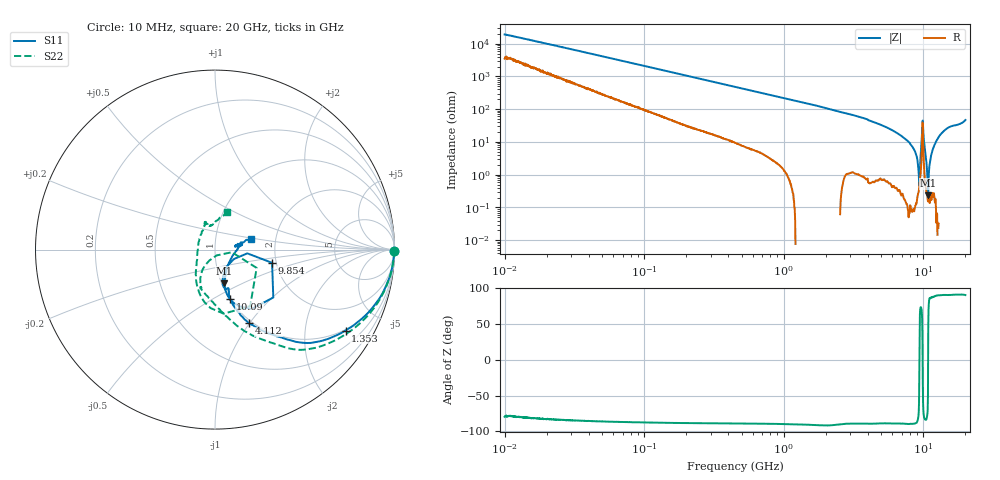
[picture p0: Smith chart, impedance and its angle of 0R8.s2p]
!Keysight Technologies,P5008B,MY61100088,A.16.20.02
!Date: Monday, October 30, 2023 15:59:24
!Correction: S11(C  2-Port  )
!S21(C  2-Port  )
!S12(C  2-Port  )
!S22(C  2-Port  )
!S2P File: Measurements: S11, S21, S12, S22:Log Frequency Sweep
# Hz S  dB  R 50
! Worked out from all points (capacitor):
!   1601 points, 10 MHz to 20 GHz, reference 50 ohm
!   read as one part in series: C = 825 fF near 10.39 MHz
!   lowest |Z| = 235 mohm at 10.84 GHz (marker M1)
!   series resonance near 9.36 GHz, so ESL is about 350 pH
!   S11 on the Smith chart (normalised r, x): 10 MHz: open; 1.353 GHz: 0.96, -3.25; 4.112 GHz: 0.96, -1.00; 9.854 GHz: 1.90, -0.31; 10.09 GHz: 1.00, -0.60; 20 GHz: 1.48, +0.18
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1e7  -0.00 -0.3  -45.63 79.2  -45.62 79.4  -0.01 -0.3
3.555162e7  -0.01 -1.0  -35.20 84.2  -35.21 84.2  -0.02 -1.1
1.263918e8  -0.04 -3.4  -24.48 84.2  -24.48 84.2  -0.04 -3.7
4.472136e8  -0.22 -11.8  -13.87 76.6  -13.87 76.6  -0.23 -12.8
8.175875e8  -0.61 -20.7  -9.15 67.8  -9.15 67.8  -0.61 -22.5
1.352781e9  -1.35 -31.8  -5.69 57.1  -5.70 57.1  -1.36 -34.7
1.589917e9  -1.73 -36.2  -4.70 53.0  -4.70 53.0  -1.73 -39.6
2.25968e9  -3.07 -47.5  -2.81 41.3  -2.81 41.3  -3.10 -52.3
4.111527e9  -6.88 -65.1  -1.04 20.4  -1.04 20.4  -6.91 -72.9
5.652411e9  -9.67 -71.7  -0.52 9.4  -0.52 9.4  -9.74 -87.2
8.750704e9  -13.54 -77.0  -0.18 -5.9  -0.19 -5.9  -13.71 -113.3
9.220141e9  -14.62 -76.7  -0.15 -8.4  -0.15 -8.4  -14.83 -117.0
9.441767e9  -15.63 -74.7  -0.14 -10.2  -0.15 -10.2  -16.04 -119.2
9.854205e9  -9.72 -13.0  -2.90 -20.1  -2.90 -20.2  -11.91 -23.8
1.009107e10  -10.82 -73.2  -0.51 -4.1  -0.52 -4.1  -11.06 -105.3
1.023592e10  -12.13 -75.3  -0.30 -6.5  -0.31 -6.5  -12.27 -112.4
1.083639e10  -14.19 -74.4  -0.15 -10.4  -0.15 -10.5  -14.23 -123.0
1.2437e10  -18.91 -50.7  -0.02 -16.4  -0.02 -16.5  -19.51 -160.2
1.298028e10  -19.80 -31.6  -0.01 -18.6  -0.01 -18.6  -20.34 172.1
1.584659e10  -16.32 12.1  -0.08 -29.5  -0.08 -29.5  -15.84 109.3
1.844831e10  -18.80 11.1  -0.07 -39.1  -0.07 -39.1  -17.16 97.4
2e10  -13.66 16.2  -0.20 -46.7  -0.20 -46.7  -13.25 72.5
